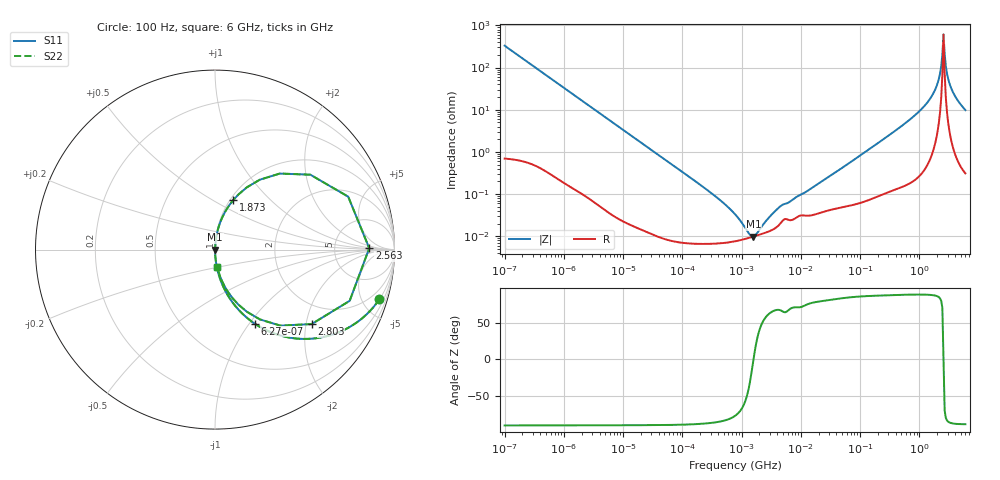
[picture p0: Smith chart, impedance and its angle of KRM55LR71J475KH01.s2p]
!Murata Part Number: KRM55LR71J475KH01
!These Parameters are Measured in Series Mode Connection
!Data Generated on Jan 08, 2026
!  o--ll--o
!Port1  Port2
!  o------o
!Operation Temp=25[degC], DC Bias Voltage=0[V]
!Freq. Start=100[Hz] Stop=6[GHz] 401[Steps]
# Hz S RI R 50
!Freq.(Hz) S11(Real) S11(Imag) S21(Real) S21(Imag) S12(Real) S12(Imag) S22(Real) S22(Imag)
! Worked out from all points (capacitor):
!   401 points, 100 Hz to 6 GHz, reference 50 ohm
!   read as one part in series: C = 4.8 uF near 109 Hz
!   lowest |Z| = 9.83 mohm at 1.586 MHz (marker M1)
!   series resonance near 1.59 MHz, so ESL is about 2.1 nH
!   S11 on the Smith chart (normalised r, x): 100 Hz: 1.01, -6.63; 627 Hz: 1.01, -1.06; 1.873 GHz: 1.03, +0.62; 2.563 GHz: 13, +1; 2.803 GHz: 1.40, -2.15; 6 GHz: 1.01, -0.20
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100  0.9161 -0.2762  0.0839 0.2762  0.0839 0.2762  0.9161 -0.2762
280  0.5842 -0.4907  0.4158 0.4907  0.4158 0.4907  0.5842 -0.4907
627  0.2215 -0.4126  0.7785 0.4126  0.7785 0.4126  0.2215 -0.4126
2008  0.0279 -0.1618  0.9721 0.1618  0.9721 0.1618  0.0279 -0.1618
40335  0.000166 -0.00838  0.9998 0.00838  0.9998 0.00838  0.000166 -0.00838
316350  6.73e-05 -0.00102  0.9999 0.00102  0.9999 0.00102  6.73e-05 -0.00102
774597  7.59e-05 -0.000325  0.9999 0.000325  0.9999 0.000325  7.59e-05 -0.000325
1325623  9.13e-05 -7.35e-05  0.9999 7.35e-05  0.9999 7.35e-05  9.13e-05 -7.35e-05
1585629  9.83e-05 -1e-06  0.9999 1e-06  0.9999 1e-06  9.83e-05 -1e-06
4440638  0.000196 0.000464  0.9998 -0.000464  0.9998 -0.000464  0.000196 0.000464
1.555665e7  0.000318 0.00138  0.9997 -0.00138  0.9997 -0.00138  0.000318 0.00138
3.124326e8  0.00176 0.0251  0.9982 -0.0251  0.9982 -0.0251  0.00176 0.0251
1.046602e9  0.0123 0.0965  0.9877 -0.0965  0.9877 -0.0965  0.0123 0.0965
1.873145e9  0.1005 0.2746  0.8995 -0.2746  0.8995 -0.2746  0.1005 0.2746
2.048624e9  0.1779 0.3471  0.8221 -0.3471  0.8221 -0.3471  0.1779 0.3471
2.240541e9  0.3608 0.4237  0.6392 -0.4237  0.6392 -0.4237  0.3608 0.4237
2.34314e9  0.5311 0.4173  0.4689 -0.4173  0.4689 -0.4173  0.5311 0.4173
2.562649e9  0.8593 0.00762  0.1407 -0.00762  0.1407 -0.00762  0.8593 0.00762
2.802721e9  0.5384 -0.4148  0.4616 0.4148  0.4616 0.4148  0.5384 -0.4148
3.065283e9  0.2502 -0.389  0.7498 0.389  0.7498 0.389  0.2502 -0.389
3.505958e9  0.0992 -0.2723  0.9008 0.2723  0.9008 0.2723  0.0992 -0.2723
6e9  0.0125 -0.0965  0.9875 0.0965  0.9875 0.0965  0.0125 -0.0965
